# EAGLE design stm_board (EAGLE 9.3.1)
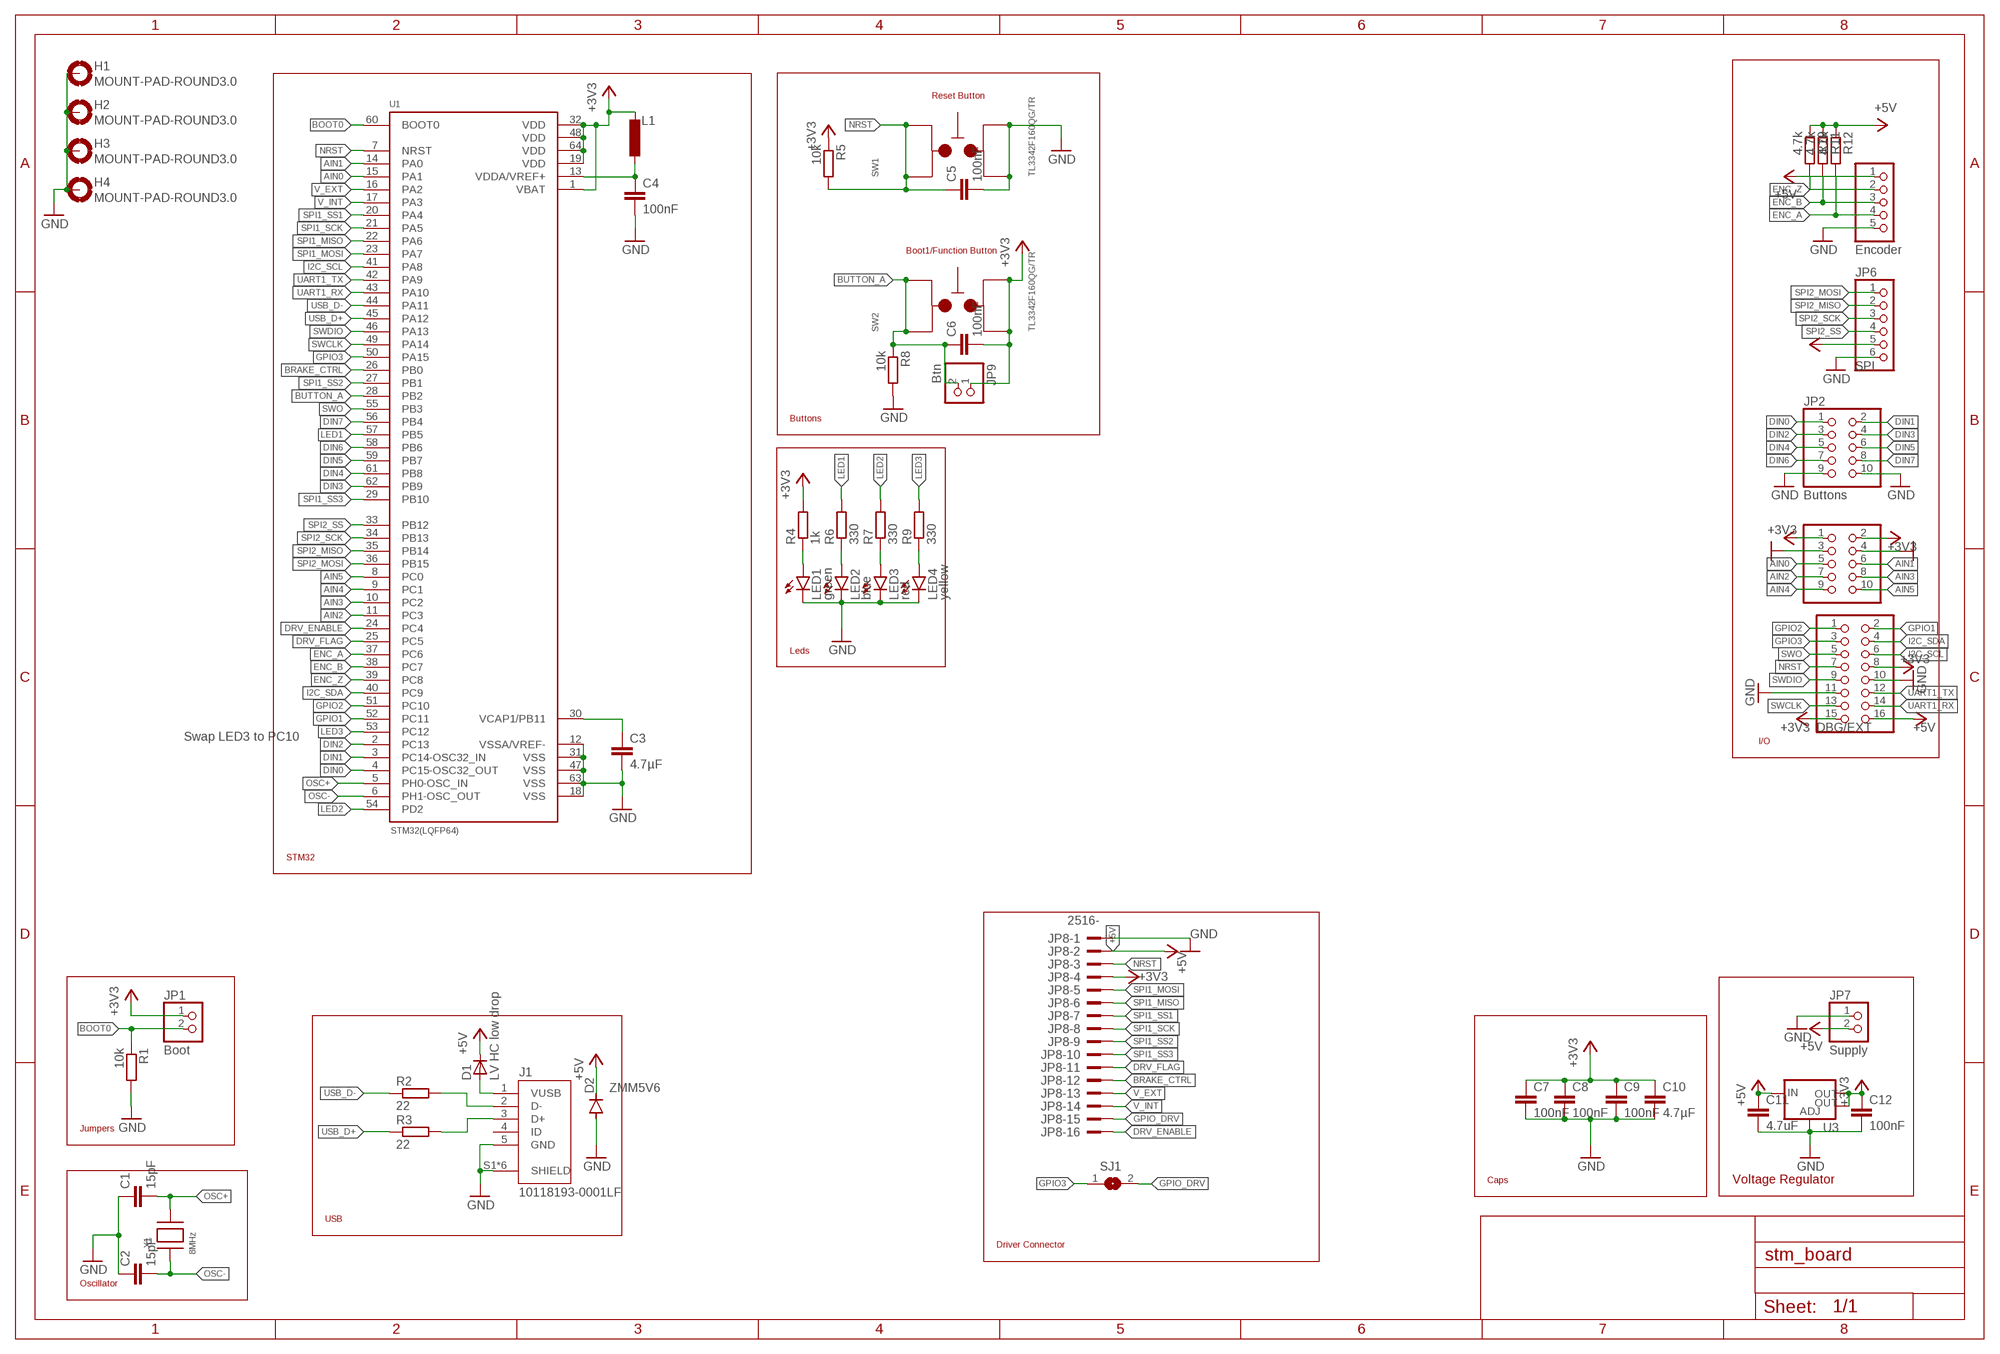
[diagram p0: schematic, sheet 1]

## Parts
C1  15pF  C-EUC0603  [C0603]
C2  15pF  C-EUC0603  [C0603]
C3  4.7µF  C-EUC0805  [C0805]
C4  100nF  C-EUC0603  [C0603]
C5  100nF  C-EUC0603  [C0603]
C6  100nF  C-EUC0603  [C0603]
C7  100nF  C-EUC0603  [C0603]
C8  100nF  C-EUC0603  [C0603]
C9  100nF  C-EUC0603  [C0603]
C10  4.7µF  C-EUC0805  [C0805]
C11  4.7uF  C-EUC0805  [C0805]
C12  100nF  C-EUC0603  [C0603]
D1  LV HC low drop  DIODESMA  [SMADIODE]
D2  ZMM5V6  DIODE-MINIMELF  [MINIMELF]
H1  MOUNT-PAD-ROUND3.0  [3,0-PAD]
H2  MOUNT-PAD-ROUND3.0  [3,0-PAD]
H3  MOUNT-PAD-ROUND3.0  [3,0-PAD]
H4  MOUNT-PAD-ROUND3.0  [3,0-PAD]
J1  10118193-0001LF  [FCI_10118193-0001LF]
JP1  Boot  PINHD-1X2  [1X02]
JP2  Buttons  PINHD-2X5  [2X05]
JP3  Analog  PINHD-2X5  [2X05]
JP4  DBG/EXT  PINHD-2X8  [2X08]
JP5  Encoder  PINHD-1X5  [1X05]
JP6  SPI  PINHD-1X6  [1X06]
JP7  Supply  PINHD-1X2  [1X02]
JP8  2516-  [PAK100/2500-16]
JP9  Btn  PINHD-1X2  [1X02]
L1  2.2µH  L-EUL2012C  [L2012C]
LED1  green  LEDCHIPLED_0805  [CHIPLED_0805]
LED2  blue  LEDCHIPLED_0805  [CHIPLED_0805]
LED3  red  LEDCHIPLED_0805  [CHIPLED_0805]
LED4  yellow  LEDCHIPLED_0805  [CHIPLED_0805]
R1  10k  R-EU_R0603  [R0603]
R2  22  R-EU_R0603  [R0603]
R3  22  R-EU_R0603  [R0603]
R4  1k  R-EU_R0603  [R0603]
R5  10k  R-EU_R0603  [R0603]
R6  330  R-EU_R0603  [R0603]
R7  330  R-EU_R0603  [R0603]
R8  10k  R-EU_R0603  [R0603]
R9  330  R-EU_R0603  [R0603]
R10  4.7k  R-EU_R0603  [R0603]
R11  4.7k  R-EU_R0603  [R0603]
R12  4.7k  R-EU_R0603  [R0603]
SJ1  SJ  [SJ]
SW1  TL3342F160QG/TR  [TL3342F160QG/TR]
SW2  TL3342F160QG/TR  [TL3342F160QG/TR]
U1  STM32(LQFP64)  [QFP50P1200X1200X160-64N]
U3  V_REG_LM1117SOT223  [SOT223]
X1  8MHz  XTALNX5032  [NX5032]

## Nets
+3V3: C6.2 C7.1 C8.1 C9.1 C10.1 C12.1 JP1.1 JP3.1 JP3.2 JP4.8 JP4.15 JP6.5 JP8.4 JP9.1 L1.1 R4.2 R5.1 SW2.1 SW2.2 U1.1(VBAT) U1.19(VDD) U1.32(VDD) U1.48(VDD) U1.64(VDD) U3.2(OUT) U3.4(OUT)
+5V: C11.1 D1.C D2.C JP4.16 JP5.1 JP7.2 JP8.2 R10.1 R11.1 R12.1 U3.3(IN)
AIN0: JP3.5 U1.15(PA1)
AIN1: JP3.6 U1.14(PA0)
AIN2: JP3.7 U1.11(PC3)
AIN3: JP3.8 U1.10(PC2)
AIN4: JP3.9 U1.9(PC1)
AIN5: JP3.10 U1.8(PC0)
BOOT0: JP1.2 R1.1 U1.60(BOOT0)
BRAKE_CTRL: JP8.12 U1.26(PB0)
BUTTON_A: C6.1 JP9.2 R8.1 SW2.3 SW2.4 U1.28(PB2)
DIN0: JP2.1 U1.4(PC15-OSC32_OUT)
DIN1: JP2.2 U1.3(PC14-OSC32_IN)
DIN2: JP2.3 U1.2(PC13)
DIN3: JP2.4 U1.62(PB9)
DIN4: JP2.5 U1.61(PB8)
DIN5: JP2.6 U1.59(PB7)
DIN6: JP2.7 U1.58(PB6)
DIN7: JP2.8 U1.56(PB4)
DRV_ENABLE: JP8.16 U1.24(PC4)
DRV_FLAG: JP8.11 U1.25(PC5)
ENC_A: JP5.4 R12.2 U1.37(PC6)
ENC_B: JP5.3 R11.2 U1.38(PC7)
ENC_Z: JP5.2 R10.2 U1.39(PC8)
GND: C1.1 C2.1 C3.2 C4.2 C5.2 C7.2 C8.2 C9.2 C10.2 C11.2 C12.2 D2.A H1.B3,0(MOUNT) H2.B3,0(MOUNT) H3.B3,0(MOUNT) H4.B3,0(MOUNT) J1.5(GND) J1.S1(SHIELD) J1.S2(SHIELD) J1.S3(SHIELD) J1.S4(SHIELD) J1.S5(SHIELD) J1.S6(SHIELD) JP2.9 JP2.10 JP3.3 JP3.4 JP4.10 JP4.11 JP5.5 JP6.6 JP7.1 JP8.1 LED1.C LED2.C LED3.C LED4.C R1.2 R8.2 SW1.1 SW1.2 U1.12(VSSA/VREF-) U1.18(VSS) U1.31(VSS) U1.47(VSS) U1.63(VSS) U3.1(ADJ)
GPIO1: JP4.2 U1.52(PC11)
GPIO2: JP4.1 U1.51(PC10)
GPIO3: JP4.3 SJ1.1 U1.50(PA15)
GPIO_DRV: JP8.15 SJ1.2
I2C_SCL: JP4.6 U1.41(PA8)
I2C_SDA: JP4.4 U1.40(PC9)
LED1: R6.2 U1.57(PB5)
LED2: R7.2 U1.54(PD2)
LED3: R9.2 U1.53(PC12)
N$1: D1.A J1.1(VUSB)
N$2: LED4.A R9.1
N$3: C4.1 L1.2 U1.13(VDDA/VREF+)
N$4: C3.1 U1.30(VCAP1/PB11)
N$5: J1.2(D-) R2.2
N$6: J1.3(D+) R3.2
N$11: LED1.A R4.1
N$12: LED2.A R6.1
N$13: LED3.A R7.1
NRST: C5.1 JP4.7 JP8.3 R5.2 SW1.3 SW1.4 U1.7(NRST)
OSC+: C1.2 U1.5(PH0-OSC_IN) X1.P$2
OSC-: C2.2 U1.6(PH1-OSC_OUT) X1.P$1
SPI1_MISO: JP8.6 U1.22(PA6)
SPI1_MOSI: JP8.5 U1.23(PA7)
SPI1_SCK: JP8.8 U1.21(PA5)
SPI1_SS1: JP8.7 U1.20(PA4)
SPI1_SS2: JP8.9 U1.27(PB1)
SPI1_SS3: JP8.10 U1.29(PB10)
SPI2_MISO: JP6.2 U1.35(PB14)
SPI2_MOSI: JP6.1 U1.36(PB15)
SPI2_SCK: JP6.3 U1.34(PB13)
SPI2_SS: JP6.4 U1.33(PB12)
SWCLK: JP4.13 U1.49(PA14)
SWDIO: JP4.9 U1.46(PA13)
SWO: JP4.5 U1.55(PB3)
UART1_RX: JP4.14 U1.43(PA10)
UART1_TX: JP4.12 U1.42(PA9)
USB_D+: R3.1 U1.45(PA12)
USB_D-: R2.1 U1.44(PA11)
V_EXT: JP8.13 U1.16(PA2)
V_INT: JP8.14 U1.17(PA3)
Unconnected: J1.4(ID)

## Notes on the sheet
- Reset Button
- Boot1/Function Button
- Buttons
- Leds
- Swap LED3 to PC10
- I/O
- STM32
- Jumpers
- Caps | Voltage Regulator
- USB
- Driver Connector
- Oscillator

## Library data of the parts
C1-C12 = resistor:C-EU: CAPACITOR, European symbol
D1 = adafruit:DIODE: Diode
D2 = diode:DIODE-: DIODE
H1-H4 = holes:MOUNT-PAD-ROUND: MOUNTING PAD, round
J1 = con_ampusb_10118193-0001LF:10118193-0001LF: Micro USB B Type Receptacle; AVAILABILITY: Unavailable; DESCRIPTION: Single Port 5 Contact Shielded SMT MICRO USB B-Type Receptacle; MF: Amphenol ICC; MP: 10118193-0001LF; PACKAGE: None; PRICE: None
JP1 JP7 JP9 = pinhead:PINHD-1X2: PIN HEADER
JP2 JP3 = pinhead:PINHD-2X5: PIN HEADER
JP4 = pinhead:PINHD-2X8: PIN HEADER
JP5 = pinhead:PINHD-1X5: PIN HEADER
JP6 = pinhead:PINHD-1X6: PIN HEADER
JP8 = con-3m:2516-: 3M (TM) Pak 100 4-Wall Header Source: 3M; OC_FARNELL: unknown; OC_NEWARK: unknown
L1 = resistor:L-EU: INDUCTOR, European symbol
LED1-LED4 = led:LED: LED
R1-R12 = resistor:R-EU_: RESISTOR, European symbol
SJ1 = jumper:SJ: SMD solder JUMPER
SW1 SW2 = Switch:TL3342F160QG/TR: SWITCH TACTILE SPST-NO 0.05A 12V Manufacturer's datasheet; CREATED_BY: PCBLayout.com; DIGI_KEY_PART_NUMBER: EG2531CT-ND; MANUFACTURER: E-Switch; MPN: TL3342F160QG/TR; PACKAGE: SPST_NO
U1 = STM32F411RET6:STM32(LQFP64); AVAILABILITY: Unavailable; MF: STMicroelectronics; MP: STM32; PACKAGE: LQFP-64 STMicroelectronics; PRICE: None
U3 = SparkFun-IC-Power:V_REG_LM1117: Voltage Regulator LM1117 Standard adjustable voltage regulator but in SMD form. Spark Fun Electronics SKU : COM-00595; PROD_ID: VREG-08170
X1 = adafruit:XTAL: Low cost SMT crystals, no capacitors included

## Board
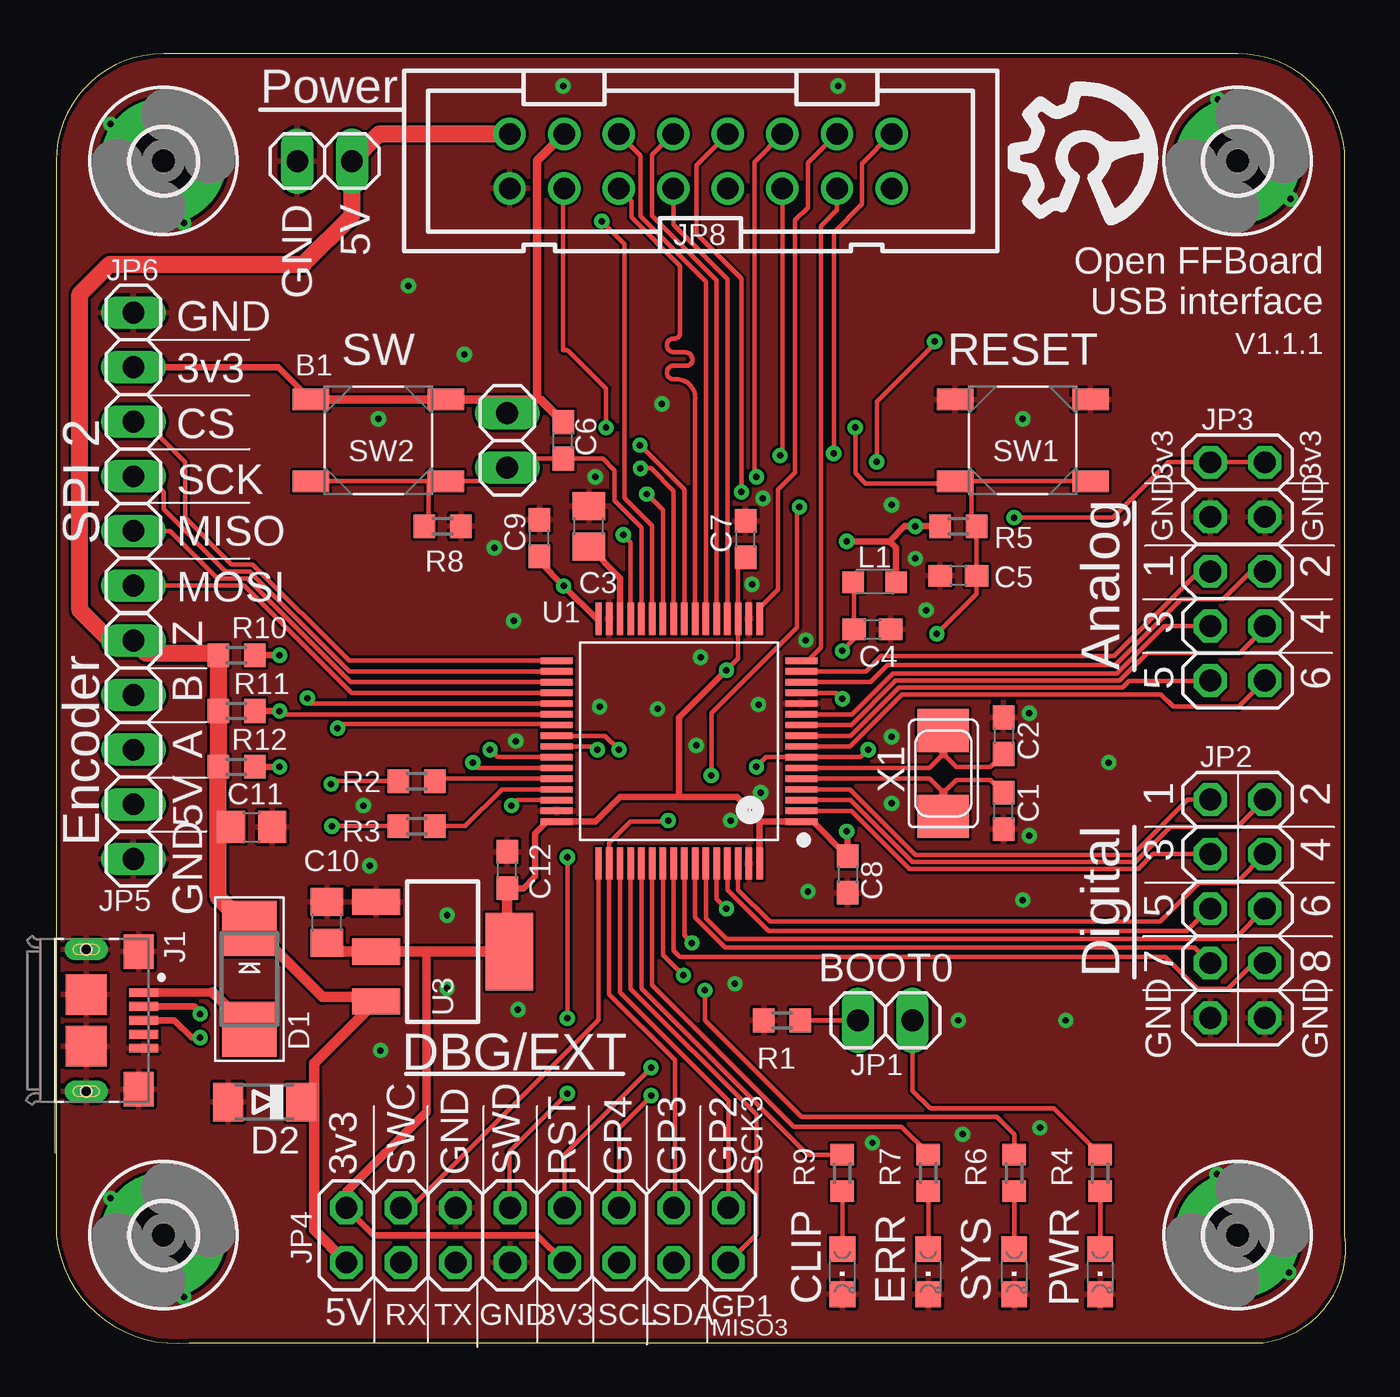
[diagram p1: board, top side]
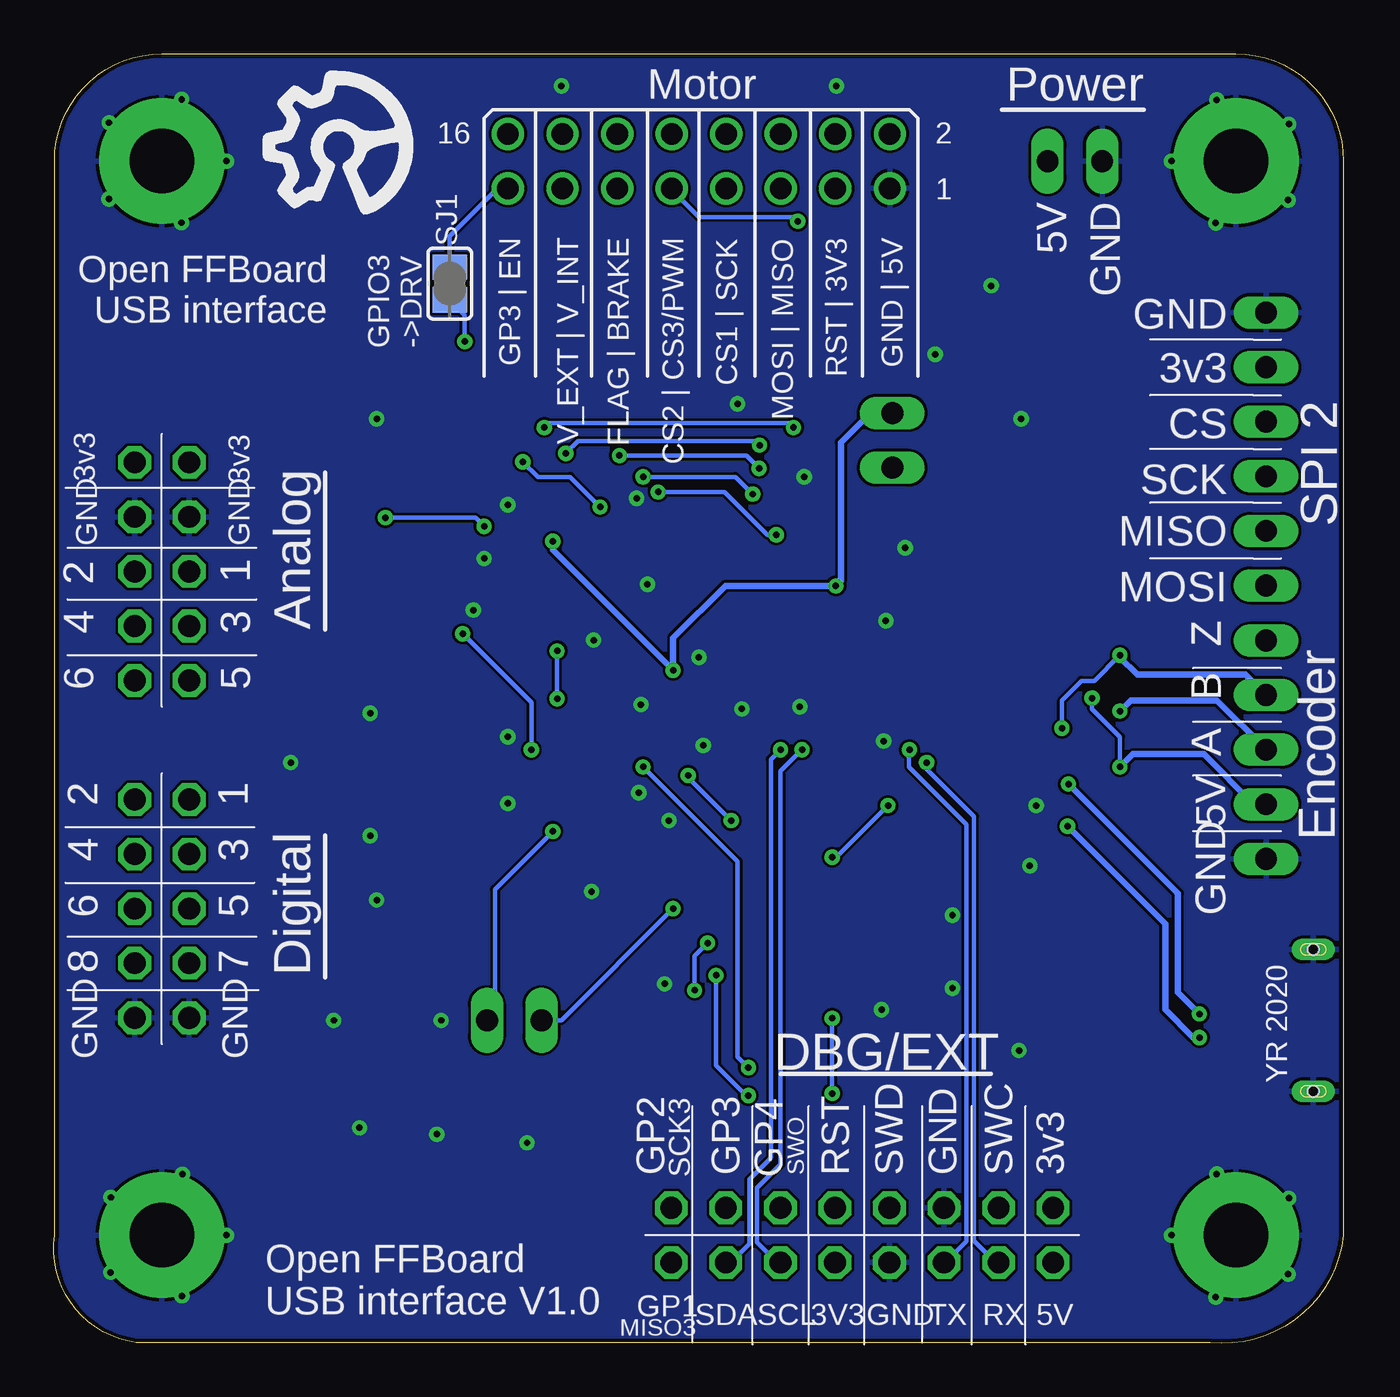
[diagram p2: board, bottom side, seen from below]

Size 60.04 x 60.03 mm. Coordinates in mm from the lower left corner, seen from the top.
Outline: 6.2,0.03 56.2,0.03 arc90 60,5.03 60,55.03 arc90 55,60.03 5,60.03 arc90 0,55.03 0,5.03 arc90 6.2,0.03
Copper layers (1*16): Top 0.035mm / dielectric 1.5mm / Bottom 0.035mm
Design rules "jlcpcb *": minimum track width 5mil, minimum drill 0.3mm, track to track 5mil, track to pad 5mil, pad to pad 5mil, via to via 5mil, smd to smd 5mil, copper to edge 0.2mm, drill to drill 8mil, minimum pad ring 10mil, minimum via ring 8mil, stop-mask expansion 2mil, vias tented up to drill 0mil, thermal gap 6mil

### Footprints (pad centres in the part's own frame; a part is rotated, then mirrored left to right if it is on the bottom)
C0603 = smd 1.1 x 1: 1 -0.85,0; 2 0.85,0
C0805 = smd 1.3 x 1.5: 1 -0.95,0; 2 0.95,0
SMADIODE = smd 2.54 x 2.54: A 2.349,0; C -2.349,0
MINIMELF = smd 1.4 x 1.8: A 1.7,0; C -1.7,0
3,0-PAD = drill 3 pad 5.842: B3,0 0,0
FCI_10118193-0001LF = smd 0.4 x 1.35: 1 -1.3,2.675; 2 -0.65,2.675; 3 0,2.675; 4 0.65,2.675; 5 1.3,2.675 | smd 1.6 x 1.4: S1 -3.2,2.45; S2 3.2,2.45 | smd 1.9 x 1.9: S3 1.2,0; S4 -1.2,0 | drill 0.5 pad 0.9 long: S5 -3.3,0; S6 3.3,0 | hole 0.5: -3.3,0; 3.3,0
1X02 = drill 1.016 long: 1 -1.27,0; 2 1.27,0
2X05 = drill 1.016 octagon: 1 -5.08,-1.27; 2 -5.08,1.27; 3 -2.54,-1.27; 4 -2.54,1.27; 5 0,-1.27; 6 0,1.27; 7 2.54,-1.27; 8 2.54,1.27; 9 5.08,-1.27; 10 5.08,1.27
2X08 = drill 1.016 octagon: 1 -8.89,-1.27; 2 -8.89,1.27; 3 -6.35,-1.27; 4 -6.35,1.27; 5 -3.81,-1.27; 6 -3.81,1.27; 7 -1.27,-1.27; 8 -1.27,1.27; 9 1.27,-1.27; 10 1.27,1.27; 11 3.81,-1.27; 12 3.81,1.27; 13 6.35,-1.27; 14 6.35,1.27; 15 8.89,-1.27; 16 8.89,1.27
1X05 = drill 1.016 long: 1 -5.08,0; 2 -2.54,0; 3 0,0; 4 2.54,0; 5 5.08,0
1X06 = drill 1.016 long: 1 -6.35,0; 2 -3.81,0; 3 -1.27,0; 4 1.27,0; 5 3.81,0; 6 6.35,0
PAK100/2500-16 = drill 1 pad 1.422: 1 -8.89,-1.27; 2 -8.89,1.27; 3 -6.35,-1.27; 4 -6.35,1.27; 5 -3.81,-1.27; 6 -3.81,1.27; 7 -1.27,-1.27; 8 -1.27,1.27; 9 1.27,-1.27; 10 1.27,1.27; 11 3.81,-1.27; 12 3.81,1.27; 13 6.35,-1.27; 14 6.35,1.27; 15 8.89,-1.27; 16 8.89,1.27
L2012C = smd 1 x 1: 1 -1,0; 2 1,0
CHIPLED_0805 = smd 1.2 x 1.2: A 0,-1.05; C 0,1.05
R0603 = smd 1 x 1.1: 1 -0.85,0; 2 0.85,0
SJ = smd 1.168 x 1.6: 1 -0.762,0; 2 0.762,0
TL3342F160QG/TR = smd 1.7 x 1: 1 -3.15,-1.9; 2 3.15,-1.9; 3 -3.15,1.9; 4 3.15,1.9
QFP50P1200X1200X160-64N = smd 1.5 x 0.3: 1 -5.7,3.75; 2 -5.7,3.25; 3 -5.7,2.75; 4 -5.7,2.25; 5 -5.7,1.75; 6 -5.7,1.25; 7 -5.7,0.75; 8 -5.7,0.25; 9 -5.7,-0.25; 10 -5.7,-0.75; 11 -5.7,-1.25; 12 -5.7,-1.75; 13 -5.7,-2.25; 14 -5.7,-2.75; 15 -5.7,-3.25; 16 -5.7,-3.75; 33 5.7,-3.75; 34 5.7,-3.25; 35 5.7,-2.75; 36 5.7,-2.25; 37 5.7,-1.75; 38 5.7,-1.25; 39 5.7,-0.75; 40 5.7,-0.25; 41 5.7,0.25; 42 5.7,0.75; 43 5.7,1.25; 44 5.7,1.75; 45 5.7,2.25; 46 5.7,2.75; 47 5.7,3.25; 48 5.7,3.75 | smd 0.3 x 1.5: 17 -3.75,-5.7; 18 -3.25,-5.7; 19 -2.75,-5.7; 20 -2.25,-5.7; 21 -1.75,-5.7; 22 -1.25,-5.7; 23 -0.75,-5.7; 24 -0.25,-5.7; 25 0.25,-5.7; 26 0.75,-5.7; 27 1.25,-5.7; 28 1.75,-5.7; 29 2.25,-5.7; 30 2.75,-5.7; 31 3.25,-5.7; 32 3.75,-5.7; 49 3.75,5.7; 50 3.25,5.7; 51 2.75,5.7; 52 2.25,5.7; 53 1.75,5.7; 54 1.25,5.7; 55 0.75,5.7; 56 0.25,5.7; 57 -0.25,5.7; 58 -0.75,5.7; 59 -1.25,5.7; 60 -1.75,5.7; 61 -2.25,5.7; 62 -2.75,5.7; 63 -3.25,5.7; 64 -3.75,5.7
SOT223 = smd 1.219 x 2.235: 1 -2.311,-3.099; 2 0,-3.099; 3 2.311,-3.099 | smd 3.6 x 2.2: 4 0,3.099
NX5032 = smd 2 x 2.4: P$1 2,0; P$2 -2,0

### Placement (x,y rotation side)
C1  44.1,24.78 90 top
C2  44.1,28.28 270 top
C3  24.8,38.03 90 top
C4  38,33.23 0 top
C5  42,35.73 180 top
C6  23.6,42.03 90 top
C7  32.1,37.43 90 top
C8  36.84,21.82 270 top
C9  22.5,37.49 90 top
C10  12.61,19.59 90 top
C11  9.1,24.03 0 top
C12  21,22.03 90 top
D1  9,16.96 270 top
D2  9.7,11.23 180 top
H1  55,5.03 0 top
H2  5,5.03 0 top
H3  55,55.03 0 top
H4  5,55.03 0 top
J1  1.4,15.03 270 top
JP1  38.6,15.03 180 top
JP2  55,20.23 270 top
JP3  55,35.93 270 top
JP4  22.4,5.03 180 top
JP5  3.6,27.63 270 top
JP6  3.6,41.63 90 top
JP7  12.5,55.03 0 top
JP8  30,55.03 0 top
JP9  21,42.03 270 top
L1  38.1,35.43 180 top
LED1  48.6,3.33 180 top
LED2  44.6,3.33 180 top
LED3  40.6,3.33 180 top
LED4  36.6,3.33 180 top
R1  33.8,15.03 180 top
R2  16.79,26.17 180 top
R3  16.79,24.07 180 top
R4  48.6,7.93 90 top
R5  42,38.03 0 top
R6  44.6,7.93 90 top
R7  40.6,7.93 90 top
R8  18,38.03 0 top
R9  36.6,7.93 90 top
R10  8.4,32.03 0 top
R11  8.4,29.43 0 top
R12  8.4,26.83 0 top
SJ1  41.6,49.33 90 bottom
SW1  45,42.03 180 top
SW2  15,42.03 180 top
U1  29,28.03 180 top
U3  18,18.23 270 top
X1  41.3,26.53 90 top

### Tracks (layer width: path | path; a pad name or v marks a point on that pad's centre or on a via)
+3V3  (via drill 0.3)
  Top 0.2: C6.2 23.6,43.23 | v31.2,31.33 31.75,31.88 U1.19 31.75,36.23 C7.1 | R4.2 46.45,10.93 40.7,10.93 39.87,11.76 JP1.1 | JP3.2 JP3.1 51.78,41.01 49.2,38.43 v44.6,38.43
  Top 0.3: 29,25.43 26.25,25.43 25.1,24.28 U1.48 22.85,24.28 22.3,23.73 22.3,21.73 21.75,21.18 C12.1 | 29,25.43 29,29.13 v31.2,31.33 | U1.32 25.2,33.68 v23.62,35.26 22.5,36.38 C9.1 | 38.8,37.33 39.5,38.03 v40,38.03 R5.1 | 38.8,37.33 v36.8,37.33 | L1.1 39.1,37.03 38.8,37.33 | 32.75,24.28 U1.1 35.23,24.28 C8.1 36.84,23.79 v36.8,23.83 | 29,25.43 31.7,25.43 32.75,24.38 32.75,24.28 | JP4.8 22.4,5.03 14.78,5.03 JP4.15 | U1.64 32.75,24.28 | JP9.1 21,43.93 | JP6.5 10.34,45.44 SW2.2
  Top 0.4: SW2.2 SW2.1 21,43.93 22.4,43.93 | 22.4,43.93 22.55,43.93 C6.2 | JP8.4 22.4,55.05 22.4,43.93 | JP4.15 13.51,7.04 17.25,10.78 17.25,18.23 16.25,18.23 16,18.23
  Top 0.5: C10.1 13.02,18.23 U3.2 16.25,18.23 | 16,18.23 U3.4 21,18.33 C12.1
  Bottom 0.2: v36.8,23.83 39.5,21.13 39.5,15.4 JP1.1 | v44.6,38.43 40.4,38.43 v40,38.03
  Bottom 0.3: v36.8,37.33 36.8,36.93 v31.2,31.33 31.2,32.83 28.77,35.26 v23.62,35.26 23.4,35.48 23.4,41.93 22,43.33 21.03,43.33 JP9.1
+5V
  Top 0.4: D2.C 12.01,11.84
  Top 0.5: R12.1 7.5,26.83 7.46,26.79 | 7.47,32.11 R10.1 | JP4.16 12,5.27 12.01,5.28 12.01,11.84 12.01,13.03 U3.3 14.71,16.11 12.4,16.11 9.98,18.54 9.98,19.31 D1.C | C11.1 7.55,24.03
  Top 0.8: R10.1 R11.1 R12.1 7.55,24.03 7.55,20.76 D1.C | 7.47,32.11 4.2,32.11 JP5.1 2.52,32.71 1.1,34.13 1.1,48.83 2.5,50.23 11.5,50.23 13.77,52.5 JP7.2 15.04,56.3 JP8.2
AIN0
  Top 0.2: U1.15 37.7,31.28 38.4,31.98 49.25,31.98 53.2,35.93 JP3.5
AIN1
  Top 0.2: U1.14 37.9,30.78 38.7,31.58 49.31,31.58 52.38,34.65 54.34,34.65 55.62,35.93 JP3.6
AIN2
  Top 0.2: U1.11 37.05,29.28 38.95,31.18 49.37,31.18 51.59,33.39 JP3.7
AIN3
  Top 0.2: U1.10 37.01,28.78 39.08,30.85 49.51,30.85 50.79,32.13 55.11,32.13 56.27,33.29 JP3.8
AIN4
  Top 0.2: U1.9 36.99,28.28 39.23,30.52 49.64,30.52 49.94,30.82 53.7,30.82 JP3.9
AIN5
  Top 0.2: U1.8 36.95,27.78 39.37,30.2 51.44,30.2 52,29.63 55.05,29.63 JP3.10
BOOT0  (via drill 0.3)
  Top 0.2: U1.60 30.75,20.68 v31.2,20.23 | JP1.2 R1.1
  Bottom 0.2: v31.2,20.23 36.4,15.03 JP1.2
BRAKE_CTRL  (via drill 0.3)
  Top 0.2: v27.5,39.53 28.25,38.78 U1.26 | JP8.12 32.5,54.99 32.5,40.43 v32.6,40.33
  Bottom 0.2: v27.5,39.53 28.3,40.33 v32.6,40.33
BUTTON_A
  Top 0.2: U1.28 27.25,37.98 26,39.23 26,40.63 25.45,41.18 C6.1 20.95,41.18 19.9,40.13 SW2.3 | SW2.3 17.35,40.13 17.35,38.23 R8.1 | SW2.3 SW2.4
  Top 0.3: JP9.2 21,41.13 20.95,41.18
DIN0
  Top 0.2: U1.4 36.95,25.78 40,22.73 50.1,22.73 52.68,25.31 JP2.1
DIN1
  Top 0.2: U1.3 36.99,25.28 39.87,22.4 50.23,22.4 51.86,24.03 54.99,24.03 JP2.2
DIN2
  Top 0.2: U1.2 37.02,24.78 39.73,22.08 50.37,22.08 51.06,22.77 JP2.3
DIN3
  Top 0.2: U1.62 31.75,21.11 33.23,19.63 51.4,19.63 53.2,21.43 54.93,21.43 JP2.4
DIN4
  Top 0.2: U1.61 31.25,21.11 33.16,19.2 52.63,19.2 53.66,20.23 JP2.5
DIN5
  Top 0.2: JP2.6 54.87,18.83 31.2,18.83 30.25,19.78 U1.59
DIN6
  Top 0.2: U1.58 29.75,19.82 31.14,18.43 52.99,18.43 JP2.7
DIN7
  Top 0.2: JP2.8 55.73,17.69 54.54,16.5 53.12,16.5 51.63,17.99 29.04,17.99 28.75,18.28 U1.56
DRV_ENABLE  (via drill 0.3)
  Top 0.2: v36.2,41.43 36.2,51.71 37.51,53.02 37.51,54.92 JP8.16 | U1.24 29.25,39.73 v27.18,41.81
  Bottom 0.2: v27.18,41.81 27.38,42.01 35.62,42.01 v36.2,41.43
DRV_FLAG  (via drill 0.3)
  Top 0.2: v27.2,40.73 27.7,40.73 28.75,39.68 U1.25 | JP8.11 33.8,41.43 v33.7,41.33
  Bottom 0.2: v33.7,41.33 27.8,41.33 v27.2,40.73
ENC_A  (via drill 0.3)
  Top 0.2: v11.7,30.03 11.7,29.83 11.75,29.78 U1.37
  Top 0.3: v10.4,26.83 R12.2
  Bottom 0.2: v10.4,26.83 10.4,28.23 11.7,29.53 v11.7,30.03
  Bottom 0.3: JP5.4 4.16,25.09 6.5,27.43 9.8,27.43 v10.4,26.83
ENC_B  (via drill 0.3)
  Top 0.2: U1.38 10.55,29.28 v10.4,29.43
  Top 0.3: v10.4,29.43 R11.2
  Bottom 0.3: JP5.3 5.9,29.93 9.9,29.93 v10.4,29.43
ENC_Z  (via drill 0.3)
  Top 0.2: U1.39 23.25,28.83 13.3,28.83 v13.1,28.63
  Top 0.3: v10.4,32.03 R10.2
  Bottom 0.2: v13.1,28.63 13.1,29.93 12.2,30.83 11.6,30.83 v10.4,32.03
  Bottom 0.3: JP5.2 4.56,31.13 9.6,31.13 10.4,31.93 v10.4,32.03
GND  (via drill 0.3)
  other vias: 45,43.03 15,43.03 28,29.53 29.8,27.83 32.8,25.63 25.3,29.63 38,9.33 42.2,9.73 42,15.03 47,15.03 18.2,19.93 18.2,16.53 19,46.03 16.4,49.23 23.6,58.53 36.4,58.53 35,21.03 45,20.63 38.9,28.23 38.9,25.13 14.6,22.23 15.1,13.63 40,36.53 38.9,39.03 32.4,35.33 28.2,43.73 21.4,28.03 20.4,37.03 25.1,40.33 34.9,32.73 32.7,29.73 32.9,39.33 14.3,25.03 45.3,29.33 45.3,23.63 52,5.03 54.05,7.87 57.38,6.8 57.39,3.3 54.06,2.21 52,55.03 54.08,57.91 57.45,56.82 57.46,53.27 54.09,52.17 8,55.03 5.94,52.15 2.57,53.21 2.54,56.75 5.89,57.88 8,5.03 5.94,2.15 2.57,3.21 2.54,6.75 5.89,7.88 31.6,16.73 30,31.93 31.4,24.33 45.8,10.03 21.3,33.63 21.5,15.53 49,27.03 40.5,34.13
  pour Top: -1,61.03 -1,-0.97 61,-0.97 61,61.03
  pour Bottom: -2,61.03 -2,-0.97 60,-0.97 60,61.03
GPIO1
  Top 0.2: U1.52 26.75,16.5 32.6,10.65 32.6,5.07 JP4.2
GPIO2
  Top 0.2: U1.51 26.25,16.33 31.29,11.29 JP4.1
GPIO3  (via drill 0.3)
  Top 0.2: v28.5,24.33 28.45,24.28 26.75,24.28 25.75,23.28 U1.50 25.75,16.23 28.8,13.18 28.8,6.35 JP4.3 | v38.2,41.03 38.2,43.83 40.9,46.53 v40.9,46.63 | v30.5,26.43 30.5,29.33 34.48,33.31 34.48,38.81 v34.6,38.93
  Bottom 0.2: v40.9,46.63 40.9,47.87 SJ1.1 | v30.5,26.43 30.5,26.33 v28.5,24.33 | v38.2,41.03 37.5,40.33 36,40.33 v34.6,38.93
GPIO_DRV
  Bottom 0.2: SJ1.2 41.6,51.53 39.37,53.76 JP8.15
I2C_SCL  (via drill 0.3)
  Top 0.2: U1.41 25.05,27.78 v25.2,27.63
  Bottom 0.2: v25.2,27.63 26.2,26.63 26.2,8.33 27.3,7.23 27.3,4.7 26.36,3.76 JP4.6
I2C_SDA  (via drill 0.3)
  Top 0.2: v26.2,27.63 25.55,28.28 U1.40
  Bottom 0.2: v26.2,27.63 26.65,27.18 26.65,8.63 27.65,7.63 27.65,4.64 28.53,3.76 JP4.4
LED1  (via drill 0.3)
  Top 0.2: R6.2 44.6,9.73 43.8,10.53 34.7,10.53 30.2,15.03 v30.2,16.43 | U1.57 29.25,18.98 v29.6,18.63
  Bottom 0.2: v29.6,18.63 30.2,18.03 v30.2,16.43
LED2
  Top 0.2: R7.2 40.6,8.83 39.35,10.08 34.35,10.08 27.75,16.68 U1.54
LED3
  Top 0.2: U1.53 27.25,16.53 35,8.78 R9.2
N$1
  Top 0.406: 7.28,16.33 J1.1
  Top 0.5: D1.A 7.28,16.33
N$2
  Top 0.2: R9.1 LED4.A
N$3  (via drill 0.3)
  Top 0.2: v36.6,30 36.32,30.28 U1.13 | v36.6,32.23 37.15,32.78 C4.1 37.15,35.38 L1.2
  Bottom 0.2: v36.6,30 v36.6,32.23
N$4
  Top 0.3: C3.1 26.25,35.63 U1.30
N$5  (via drill 0.3)
  Top 0.2: v12.8,26.03 12.94,26.17 R2.2
  Top 0.3: J1.2 6.45,15.68 6.7,15.43 v6.7,15.33
  Bottom 0.3: v6.7,15.33 7.7,16.33 7.7,20.93 v12.8,26.03
N$6  (via drill 0.3)
  Top 0.2: R3.2 v12.84,24.07
  Top 0.3: v6.7,14.23 6.3,14.23 5.5,15.03 J1.3
  Bottom 0.3: v6.7,14.23 7,14.23 8.3,15.53 8.3,19.53 v12.84,24.07
N$11
  Top 0.2: R4.1 LED1.A
N$12
  Top 0.2: R6.1 LED2.A
N$13
  Top 0.2: R7.1 LED3.A
NRST  (via drill 0.3)
  Top 0.2: v37.8,27.63 37.45,27.28 U1.7 33.05,27.28 v32.6,26.83 | 42.6,40.13 SW1.4 41.75,40.03 37.68,40.03 37.2,40.51 v37.2,42.63 | 42.6,40.13 SW1.3 | v25.6,42.63 25.6,44.43 23.8,46.23 23.6,46.23 23.6,53.71 JP8.3 | 42.6,40.13 42.6,38.28 R5.2 42.85,36.03 42.85,34.88 v41,33.03 | v27.7,12.83 23.67,8.8 JP4.7
  Top 0.3: C5.1 42.85,36.03
  Bottom 0.2: v37.8,27.63 37.8,29.83 v41,33.03 | v32.6,26.83 28.2,22.43 28.2,13.33 v27.7,12.83 | v37.2,42.63 37,42.83 25.8,42.83 v25.6,42.63
OSC+
  Top 0.2: C1.2 43.5,26.23 41.9,26.23 41.3,25.63 40.65,26.28 U1.5
  Top 0.4: X1.P$2 41.3,25.63
OSC-
  Top 0.2: U1.6 40.65,26.78 41.3,27.43 41.9,26.83 43.5,26.83 C2.2
  Top 0.4: X1.P$1 41.3,27.43
SPI1_MISO
  Top 0.2: U1.22 30.25,49.41 27.2,52.46 27.2,55.29 JP8.6
SPI1_MOSI
  Top 0.2: JP8.5 26.79,53.16 26.79,52.41 29.05,50.15 29.05,47.03 arc-90 28.79,46.77 28.75,46.77 arc90 28.43,46.46 arc90 28.75,46.14 29.25,46.14 arc-90 29.62,45.78 arc-90 29.36,45.51 28.75,45.51 arc90 28.43,45.2 arc90 28.75,44.88 28.79,44.88 arc-100 29.75,43.92 U1.23
SPI1_SCK
  Top 0.2: U1.21 30.75,49.48 27.75,52.48 27.75,55.32 JP8.8
SPI1_SS1
  Top 0.2: JP8.7 28.73,52.06 31.25,49.54 U1.20
SPI1_SS2  (via drill 0.3)
  Top 0.2: U1.27 27.75,38.06 26.46,39.35 26.46,51.17 v25.4,52.23
  Bottom 0.2: v25.4,52.23 25.6,52.43 30,52.43 31.27,53.7 JP8.9
SPI1_SS3  (via drill 0.3)
  Top 0.2: U1.29 26.75,37.28 v26.4,37.63 | v31.9,39.63 31.9,49.56 29.8,51.66 29.8,54.83 JP8.10
  Bottom 0.2: v31.9,39.63 28.8,39.63 26.8,37.63 v26.4,37.63
SPI2_MISO
  Top 0.2: U1.35 13.71,30.78 8.88,35.61 7.51,35.61 5.3,37.82 JP6.2
SPI2_MOSI
  Top 0.2: JP6.1 8.75,35.28 13.75,30.28 U1.36
SPI2_SCK
  Top 0.2: U1.34 13.68,31.28 9.02,35.94 7.9,35.94 5,38.83 5,39.63 4.27,40.36 JP6.3
SPI2_SS
  Top 0.2: U1.33 13.64,31.78 9.16,36.26 8.17,36.26 6,38.43 6,41.03 4.13,42.9 JP6.4
SWCLK
  Top 0.2: U1.49 25.25,15.05 16.5,6.3 JP4.13
SWDIO  (via drill 0.3)
  Top 0.2: U1.46 21.45,25.28 v21.2,25.03 | v23.8,22.63 v23.8,15.13 | JP4.9 21.1,6.33 21.1,8.93 v23.8,11.63
  Bottom 0.2: v23.8,15.13 v23.8,11.63 | v21.2,25.03 23.6,22.63 v23.8,22.63
SWO  (via drill 0.3)
  Top 0.2: U1.55 28.25,18.08 v29.2,17.13 | JP4.5 26.21,10 27.7,11.49 v27.7,11.53
  Bottom 0.2: v29.2,17.13 29.2,12.93 27.8,11.53 v27.7,11.53
UART1_RX  (via drill 0.3)
  Top 0.2: U1.43 19.65,26.78 v19.4,27.03
  Bottom 0.2: v19.4,27.03 19.4,26.73 17.2,24.53 17.2,4.77 16.19,3.76 JP4.14
UART1_TX  (via drill 0.3)
  Top 0.2: U1.42 20.55,27.28 v20.2,27.63
  Bottom 0.2: v20.2,27.63 20.21,27.62 20.21,26.83 17.54,24.16 17.54,4.75 18.53,3.76 JP4.12
USB_D+
  Top 0.2: U1.45 20.75,25.78 19.04,24.07 R3.1
USB_D-
  Top 0.2: U1.44 17.64,26.28 R2.1
V_EXT
  Top 0.2: U1.16 35,31.78 35.6,32.38 35.6,52.01 36.35,52.76 JP8.13
V_INT
  Top 0.2: U1.17 32.75,34.23 33.6,35.08 33.6,39.73 34.4,40.53 34.4,52.27 35,52.87 35,54.95 JP8.14

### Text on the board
tPlace: Power | GND | 5V | Open FFBoard / USB interface | GND | V1.1.1 | B1 | SW | RESET | 3v3 | SPI 2 | CS | SCK | 3v3 | 3v3 | MISO | GND | GND | 1 | 2 | MOSI | 3 | 4 | Encoder | Z | Analog | B | 5 | 6 | A | 1 | 2 | 5V | 3 | 4 | GND | 5 | 6 | BOOT0 | Digital | 7 | 8 | DBG/EXT | GND | GND | 3v3 | SWC | GND | SWD | RST | GP4 | GP3 | GP2 | SCK3 | CLIP | ERR | SYS | PWR | 5V | RX | TX | GND | 3V3 | SCL | SDA | GP1 | MISO3
bPlace: Power | Motor | 2 | 16 | GND | 5V | 1 | GND | 5V | RST | 3V3 | MOSI | MISO | CS1 | SCK | CS2 | CS3/PWM | FLAG | BRAKE | V_EXT | V_INT | GP3 | EN | Open FFBoard / USB interface | GND | 3v3 | GPIO3 / ->DRV | CS | SCK | 3v3 | 3v3 | SPI 2 | MISO | GND | GND | MOSI | 1 | 2 | Analog | 3 | 4 | Z | B | 5 | 6 | A | 1 | 2 | 5V | Encoder | 3 | 4 | GND | 5 | 6 | Digital | 7 | 8 | DBG/EXT | GND | GND | YR 2020 | 3v3 | SWC | GND | SWD | RST | SWO | GP4 | GP3 | SCK3 | GP2 | 5V | RX | TX | GND | 3V3 | SCL | SDA | GP1 | Open FFBoard / USB interface V1.0 | MISO3
tDocu: JLCJLCJLCJLC

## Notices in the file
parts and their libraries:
SparkFun-IC-Power: Licensing: Creative Commons ShareAlike 4.0 International - https://creativecommons.org/licenses/by-sa/4.0
